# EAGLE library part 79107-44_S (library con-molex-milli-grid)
RECEPTACAL
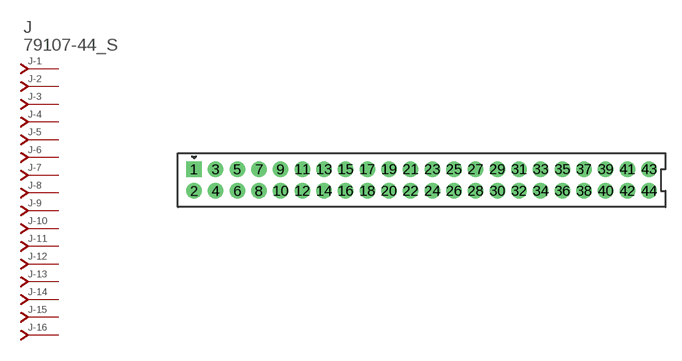
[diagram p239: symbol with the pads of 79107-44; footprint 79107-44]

Designator prefix J; gates -1=J-NV -2=J-N -3=J-N -4=J-N -5=J-N -6=J-N -7=J-N -8=J-N -9=J-N -10=J-N -11=J-N -12=J-N -13=J-N -14=J-N -15=J-N -16=J-N -17=J-N -18=J-N -19=J-N -20=J-N -21=J-N -22=J-N -23=J-N -24=J-N -25=J-N -26=J-N -27=J-N -28=J-N -29=J-N -30=J-N -31=J-N -32=J-N -33=J-N -34=J-N -35=J-N -36=J-N -37=J-N -38=J-N -39=J-N -40=J-N -41=J-N -42=J-N -43=J-N -44=J-N

## 79107-44_S  [79107-44]
1  -1:J  pas
2  -2:J  pas
3  -3:J  pas
4  -4:J  pas
5  -5:J  pas
6  -6:J  pas
7  -7:J  pas
8  -8:J  pas
9  -9:J  pas
10  -10:J  pas
11  -11:J  pas
12  -12:J  pas
13  -13:J  pas
14  -14:J  pas
15  -15:J  pas
16  -16:J  pas
17  -17:J  pas
18  -18:J  pas
19  -19:J  pas
20  -20:J  pas
21  -21:J  pas
22  -22:J  pas
23  -23:J  pas
24  -24:J  pas
25  -25:J  pas
26  -26:J  pas
27  -27:J  pas
28  -28:J  pas
29  -29:J  pas
30  -30:J  pas
31  -31:J  pas
32  -32:J  pas
33  -33:J  pas
34  -34:J  pas
35  -35:J  pas
36  -36:J  pas
37  -37:J  pas
38  -38:J  pas
39  -39:J  pas
40  -40:J  pas
41  -41:J  pas
42  -42:J  pas
43  -43:J  pas
44  -44:J  pas

## Footprint 79107-44 (pad centres in mm)
RECEPTACAL Dual Row, Vertical, Through-Hole
drill 0.914 square: 1 -21,1
drill 0.914: 2 -21,-1; 3 -19,1; 4 -19,-1; 5 -17,1; 6 -17,-1; 7 -15,1; 8 -15,-1; 9 -13,1; 10 -13,-1; 11 -11,1; 12 -11,-1; 13 -9,1; 14 -9,-1; 15 -7,1; 16 -7,-1; 17 -5,1; 18 -5,-1; 19 -3,1; 20 -3,-1; 21 -1,1; 22 -1,-1; 23 1,1; 24 1,-1; 25 3,1; 26 3,-1; 27 5,1; 28 5,-1; 29 7,1; 30 7,-1; 31 9,1; 32 9,-1; 33 11,1; 34 11,-1; 35 13,1; 36 13,-1; 37 15,1; 38 15,-1; 39 17,1; 40 17,-1; 41 19,1; 42 19,-1; 43 21,1; 44 21,-1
